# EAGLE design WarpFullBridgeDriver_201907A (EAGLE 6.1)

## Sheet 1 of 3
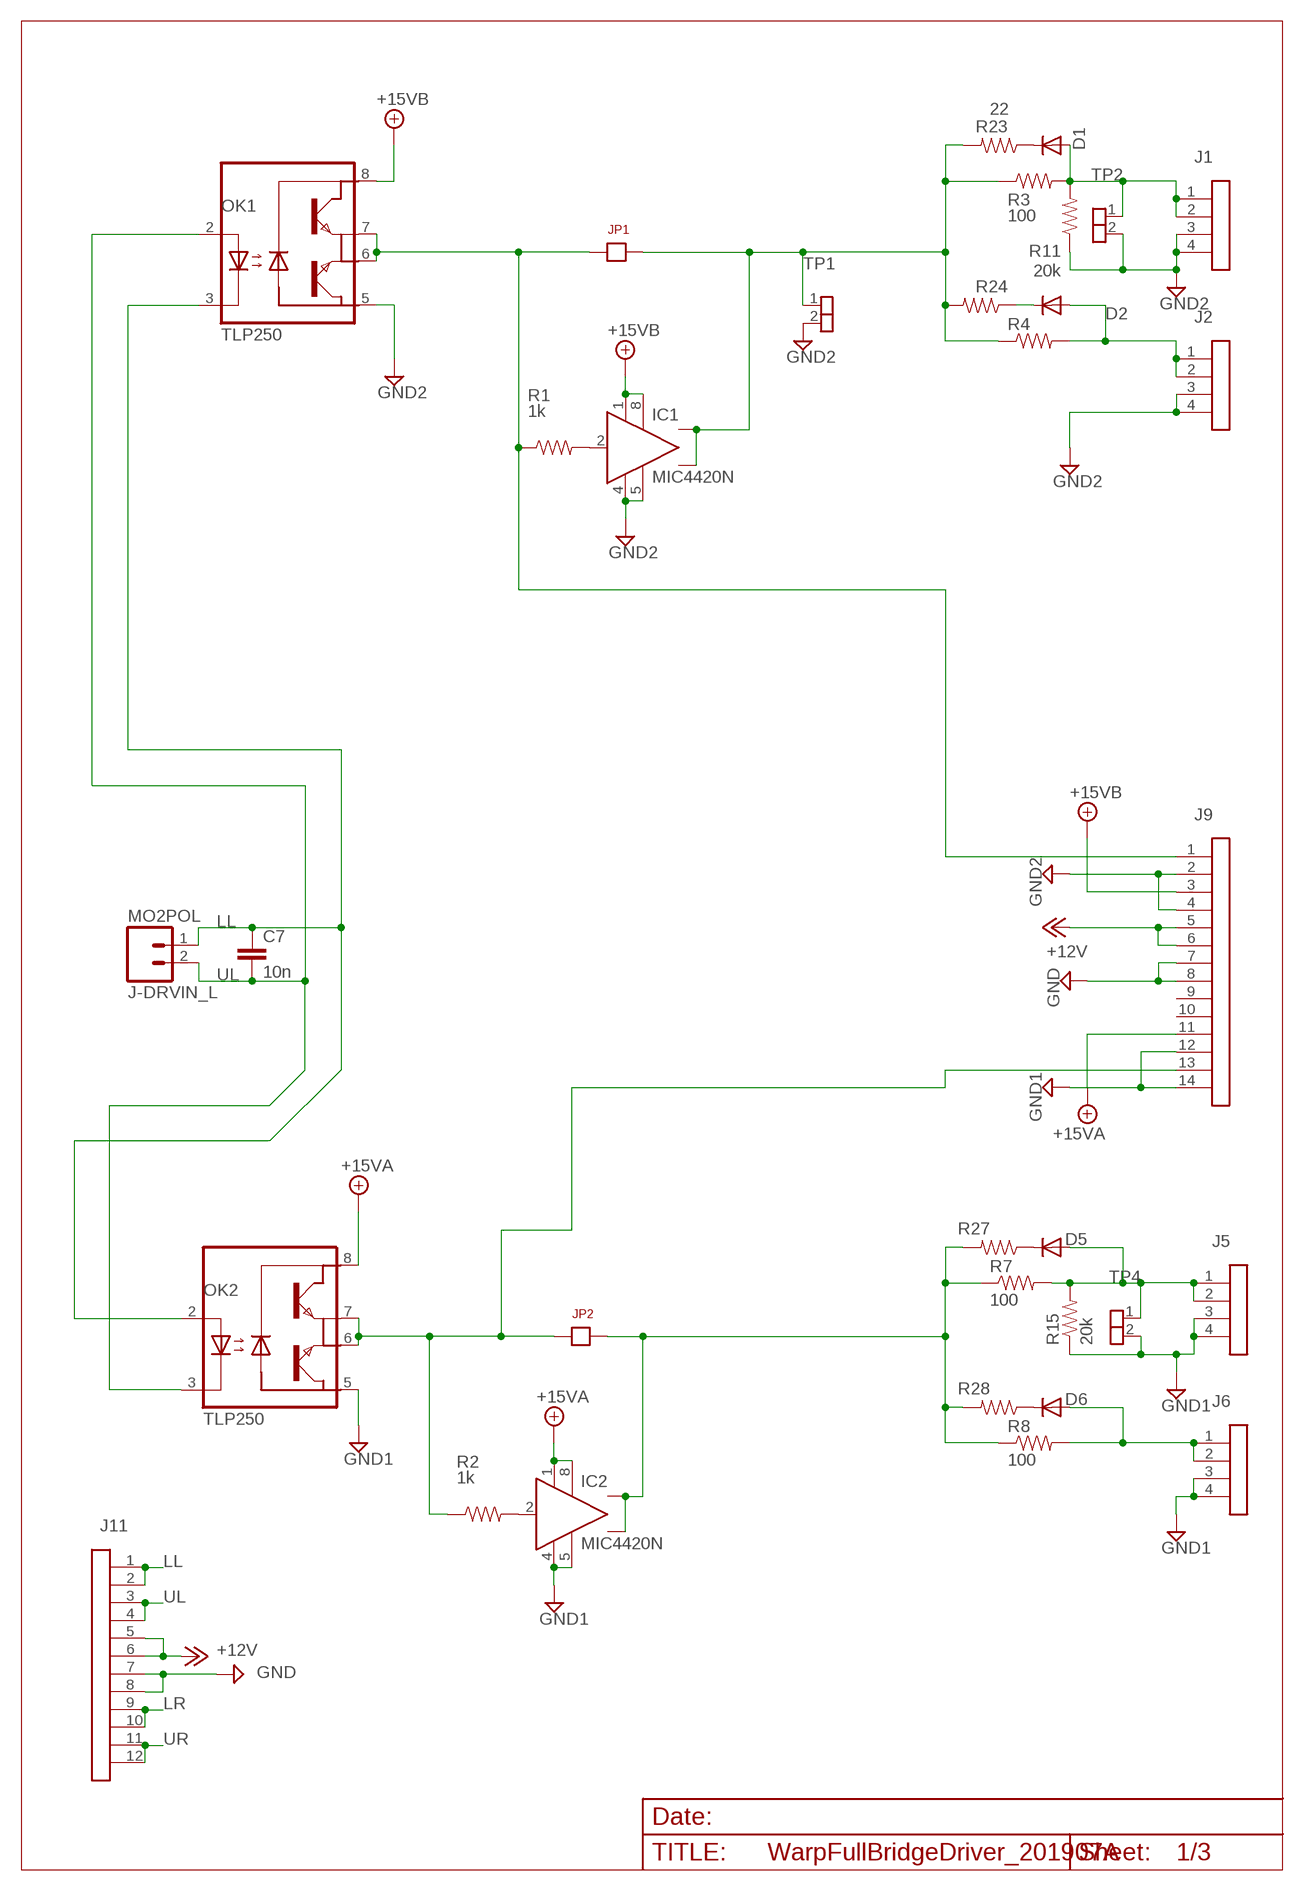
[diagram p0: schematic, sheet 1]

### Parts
C7  10n  BCAP  [BCAP]
D1  1N4148DO35-7  [D3]
D2  1N4148DO35-7  [D3]
D5  1N4148DO35-7  [D3]
D6  1N4148DO35-7  [D3]
IC1  MIC4420N  [DIL08]
IC2  MIC4420N  [DIL08]
J1  IDC04  [IDC04]
J2  IDC04  [IDC04]
J5  IDC04  [IDC04]
J6  IDC04  [IDC04]
J9  IDC14_LSPECIAL1  [IDC14-SPECIAL]
J11  IDC12  [IDC12]
J-DRVIN_L  MO2POL  [MOLEX-1X2]
JP1  JP1  [JP1]
JP2  JP1  [JP1]
OK1  TLP250  TLP250DIP8-L39  [DIL08-L39]
OK2  TLP250  TLP250DIP8-L39  [DIL08-L39]
R1  1k  RESISTORPTH-1/4W  [AXIAL-0.4]
R2  1k  RESISTORPTH-1/4W  [AXIAL-0.4]
R3  100  RESISTORPTH-1/4W  [AXIAL-0.4]
R4  100  RESISTORPTH-1/4W  [AXIAL-0.4]
R7  100  RESISTORPTH-1/4W  [AXIAL-0.4]
R8  100  RESISTORPTH-1/4W  [AXIAL-0.4]
R11  20k  R4  [AXIAL-0.4]
R15  20k  R4  [AXIAL-0.4]
R23  22  R4  [AXIAL-0.4]
R24  22  R4  [AXIAL-0.4]
R27  22  R4  [AXIAL-0.4]
R28  22  R4  [AXIAL-0.4]
TP1  SIL-2  [JP1]
TP2  SIL-2  [JP1]
TP4  SIL-2  [JP1]

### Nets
+12V: J9.5 J9.6 J11.5 J11.6 ; also sheet 2,3
+15VA: IC2.1(VS) IC2.8(VS1) J9.11 OK2.8(VCC) ; also sheet 3
+15VB: IC1.1(VS) IC1.8(VS1) J9.3 OK1.8(VCC) ; also sheet 3
GND: J9.7 J9.8 J11.7 J11.8 ; also sheet 2,3
GND1: IC2.4(GND) IC2.5(GND1) J5.3 J5.4 J6.3 J6.4 J9.12 J9.14 OK2.5(GND) R15.P$1 TP4.2 ; also sheet 3
GND2: IC1.4(GND) IC1.5(GND1) J1.3 J1.4 J2.3 J2.4 J9.2 J9.4 OK1.5(GND) R11.P$1 TP1.2 TP2.2 ; also sheet 3
LL: C7.1 J11.1 J11.2 J-DRVIN_L.1 OK1.3(C) OK2.2(A)
LR: J11.9 J11.10 ; also sheet 2
N$2: D2.A J2.1 J2.2 R4.P$2
N$3: D1.A J1.1 J1.2 R3.P$2 R11.P$2 TP2.1
N$4: D1.C R23.P$1
N$5: IC1.2(IN) R1.P$2
N$7: IC2.2(IN) R2.P$2
N$8: D6.A J6.1 J6.2 R8.P$2
N$12: D5.A J5.1 J5.2 R7.P$2 R15.P$2 TP4.1
N$17: IC1.6(OUT) IC1.7(OUT) JP1.2 R3.P$1 R4.P$1 R23.P$2 R24.P$2 TP1.1
N$18: J9.1 JP1.1 OK1.6(VO) OK1.7(VO2) R1.P$1
N$19: IC2.6(OUT) IC2.7(OUT) JP2.2 R7.P$1 R8.P$1 R27.P$2 R28.P$2
N$21: D2.C R24.P$1
N$22: J9.13 JP2.1 OK2.6(VO) OK2.7(VO2) R2.P$1
N$28: D5.C R27.P$1
N$31: D6.C R28.P$1
UL: C7.2 J11.3 J11.4 J-DRVIN_L.2 OK1.2(A) OK2.3(C)
UR: J11.11 J11.12 ; also sheet 2
Unconnected: J9.9 J9.10

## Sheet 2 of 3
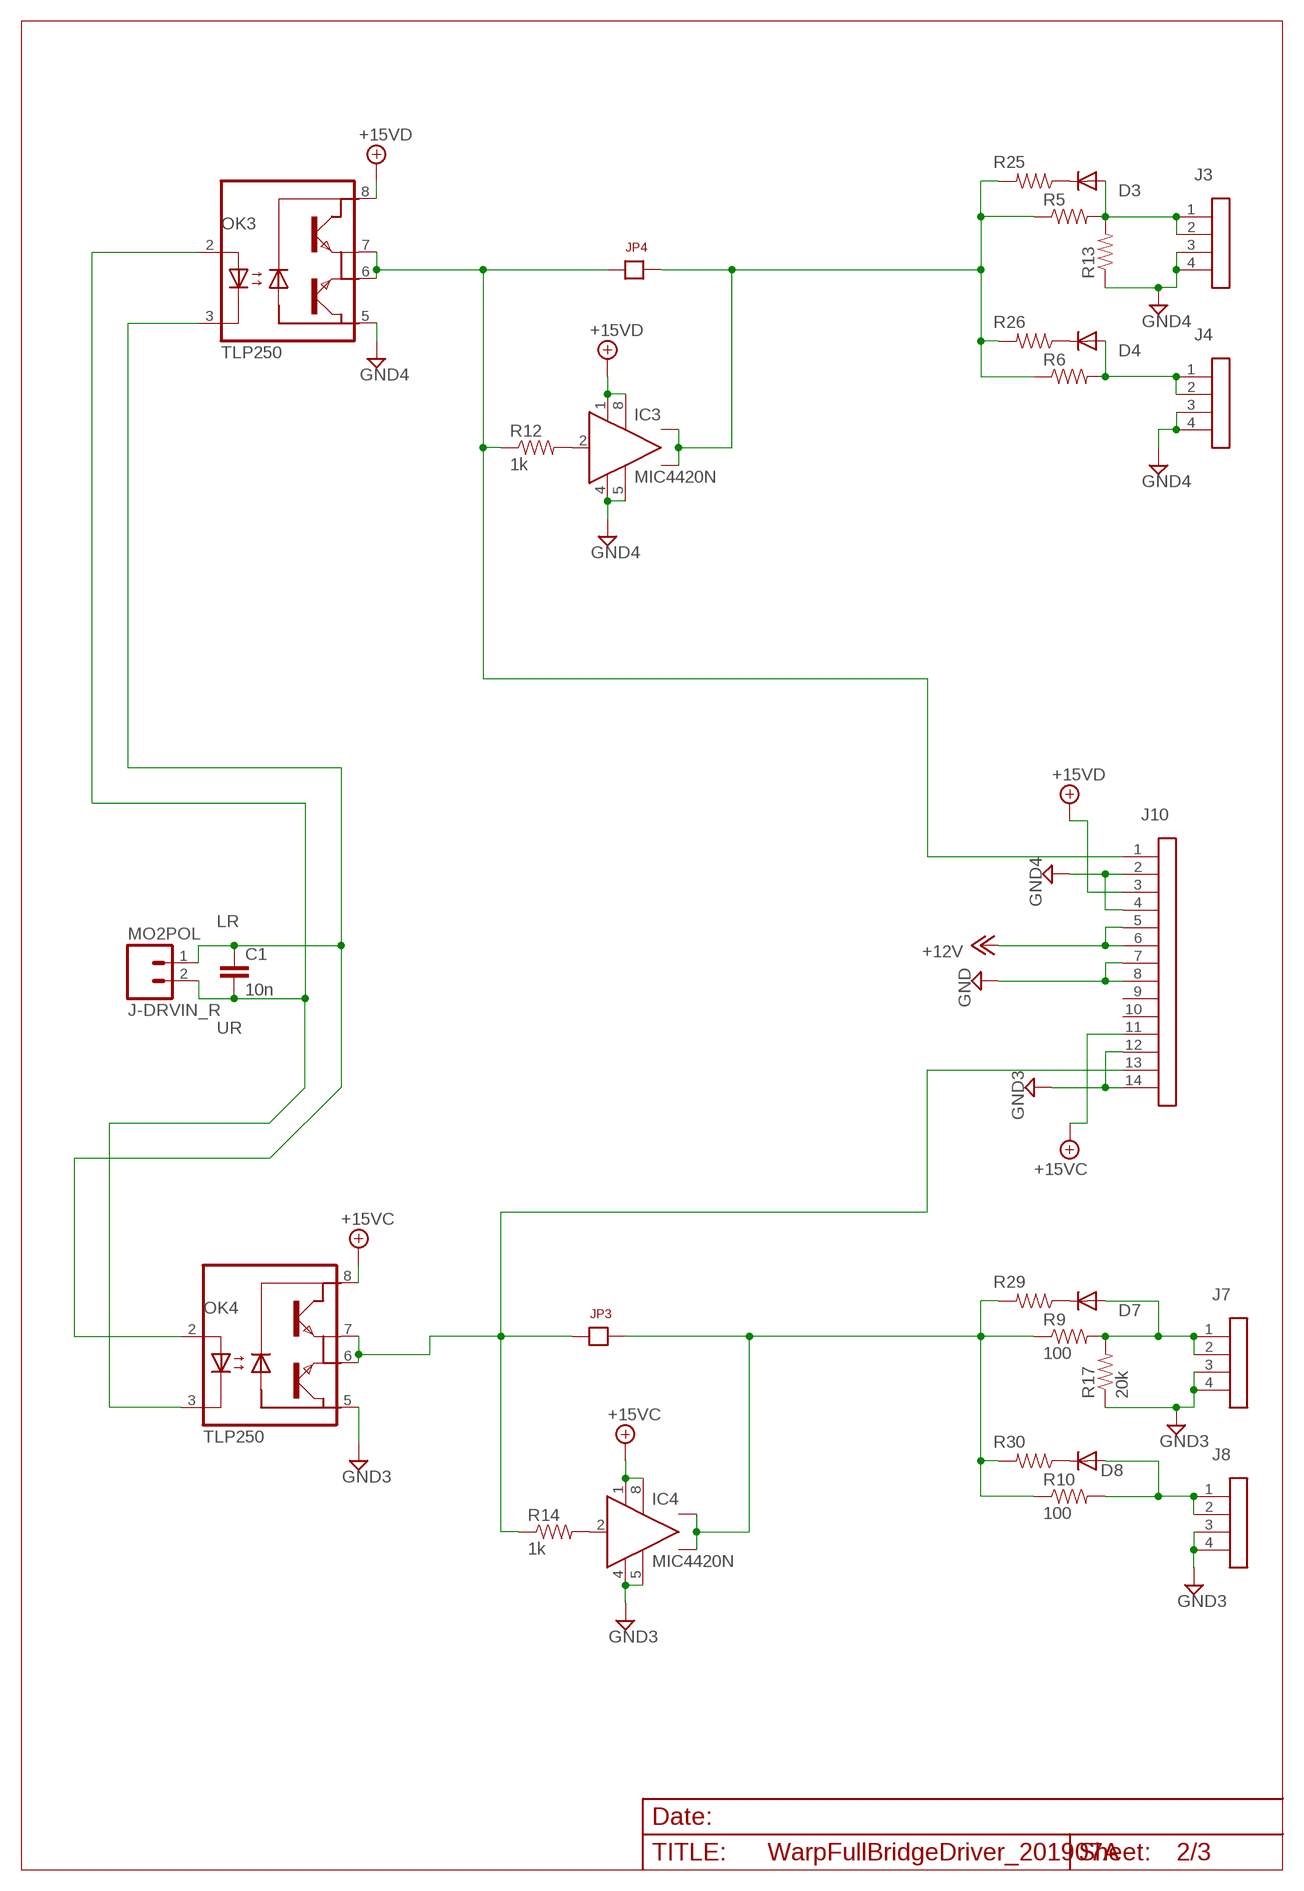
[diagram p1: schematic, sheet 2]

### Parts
C1  10n  BCAP  [BCAP]
D3  1N4148DO35-7  [D3]
D4  1N4148DO35-7  [D3]
D7  1N4148DO35-7  [D3]
D8  1N4148DO35-7  [D3]
IC3  MIC4420N  [DIL08]
IC4  MIC4420N  [DIL08]
J3  IDC04  [IDC04]
J4  IDC04  [IDC04]
J7  IDC04  [IDC04]
J8  IDC04  [IDC04]
J10  IDC14_LSPECIAL1  [IDC14-SPECIAL]
J-DRVIN_R  MO2POL  [MOLEX-1X2]
JP3  JP1  [JP1]
JP4  JP1  [JP1]
OK3  TLP250  TLP250DIP8-L39  [DIL08-L39]
OK4  TLP250  TLP250DIP8-L39  [DIL08-L39]
R5  100  RESISTORPTH-1/4W  [AXIAL-0.4]
R6  100  RESISTORPTH-1/4W  [AXIAL-0.4]
R9  100  RESISTORPTH-1/4W  [AXIAL-0.4]
R10  100  RESISTORPTH-1/4W  [AXIAL-0.4]
R12  1k  R4  [AXIAL-0.4]
R13  20k  R4  [AXIAL-0.4]
R14  1k  R4  [AXIAL-0.4]
R17  20k  R4  [AXIAL-0.4]
R25  22  R4  [AXIAL-0.4]
R26  22  R4  [AXIAL-0.4]
R29  22  R4  [AXIAL-0.4]
R30  22  R4  [AXIAL-0.4]

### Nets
+12V: J10.5 J10.6 ; also sheet 1,3
+15VC: IC4.1(VS) IC4.8(VS1) J10.11 OK4.8(VCC) ; also sheet 3
+15VD: IC3.1(VS) IC3.8(VS1) J10.3 OK3.8(VCC) ; also sheet 3
GND: J10.7 J10.8 ; also sheet 1,3
GND3: IC4.4(GND) IC4.5(GND1) J7.3 J7.4 J8.3 J8.4 J10.12 J10.14 OK4.5(GND) R17.P$1 ; also sheet 3
GND4: IC3.4(GND) IC3.5(GND1) J3.3 J3.4 J4.3 J4.4 J10.2 J10.4 OK3.5(GND) R13.P$1 ; also sheet 3
LR: C1.1 J-DRVIN_R.1 OK3.3(C) OK4.2(A) ; also sheet 1
N$1: IC3.6(OUT) IC3.7(OUT) JP4.2 R5.P$1 R6.P$1 R25.P$2 R26.P$2
N$6: IC4.6(OUT) IC4.7(OUT) JP3.2 R9.P$1 R10.P$1 R29.P$2 R30.P$2
N$9: D3.A J3.1 J3.2 R5.P$2 R13.P$2
N$10: D4.A J4.1 J4.2 R6.P$2
N$11: IC3.2(IN) R12.P$2
N$13: D7.A J7.1 J7.2 R9.P$2 R17.P$2
N$14: D8.A J8.1 J8.2 R10.P$2
N$15: J10.1 JP4.1 OK3.6(VO) OK3.7(VO2) R12.P$1
N$16: IC4.2(IN) R14.P$2
N$24: D3.C R25.P$1
N$25: D4.C R26.P$1
N$33: J10.13 JP3.1 OK4.6(VO) OK4.7(VO2) R14.P$1
N$34: D7.C R29.P$1
N$37: D8.C R30.P$1
UR: C1.2 J-DRVIN_R.2 OK3.2(A) OK4.3(C) ; also sheet 1
Unconnected: J10.9 J10.10

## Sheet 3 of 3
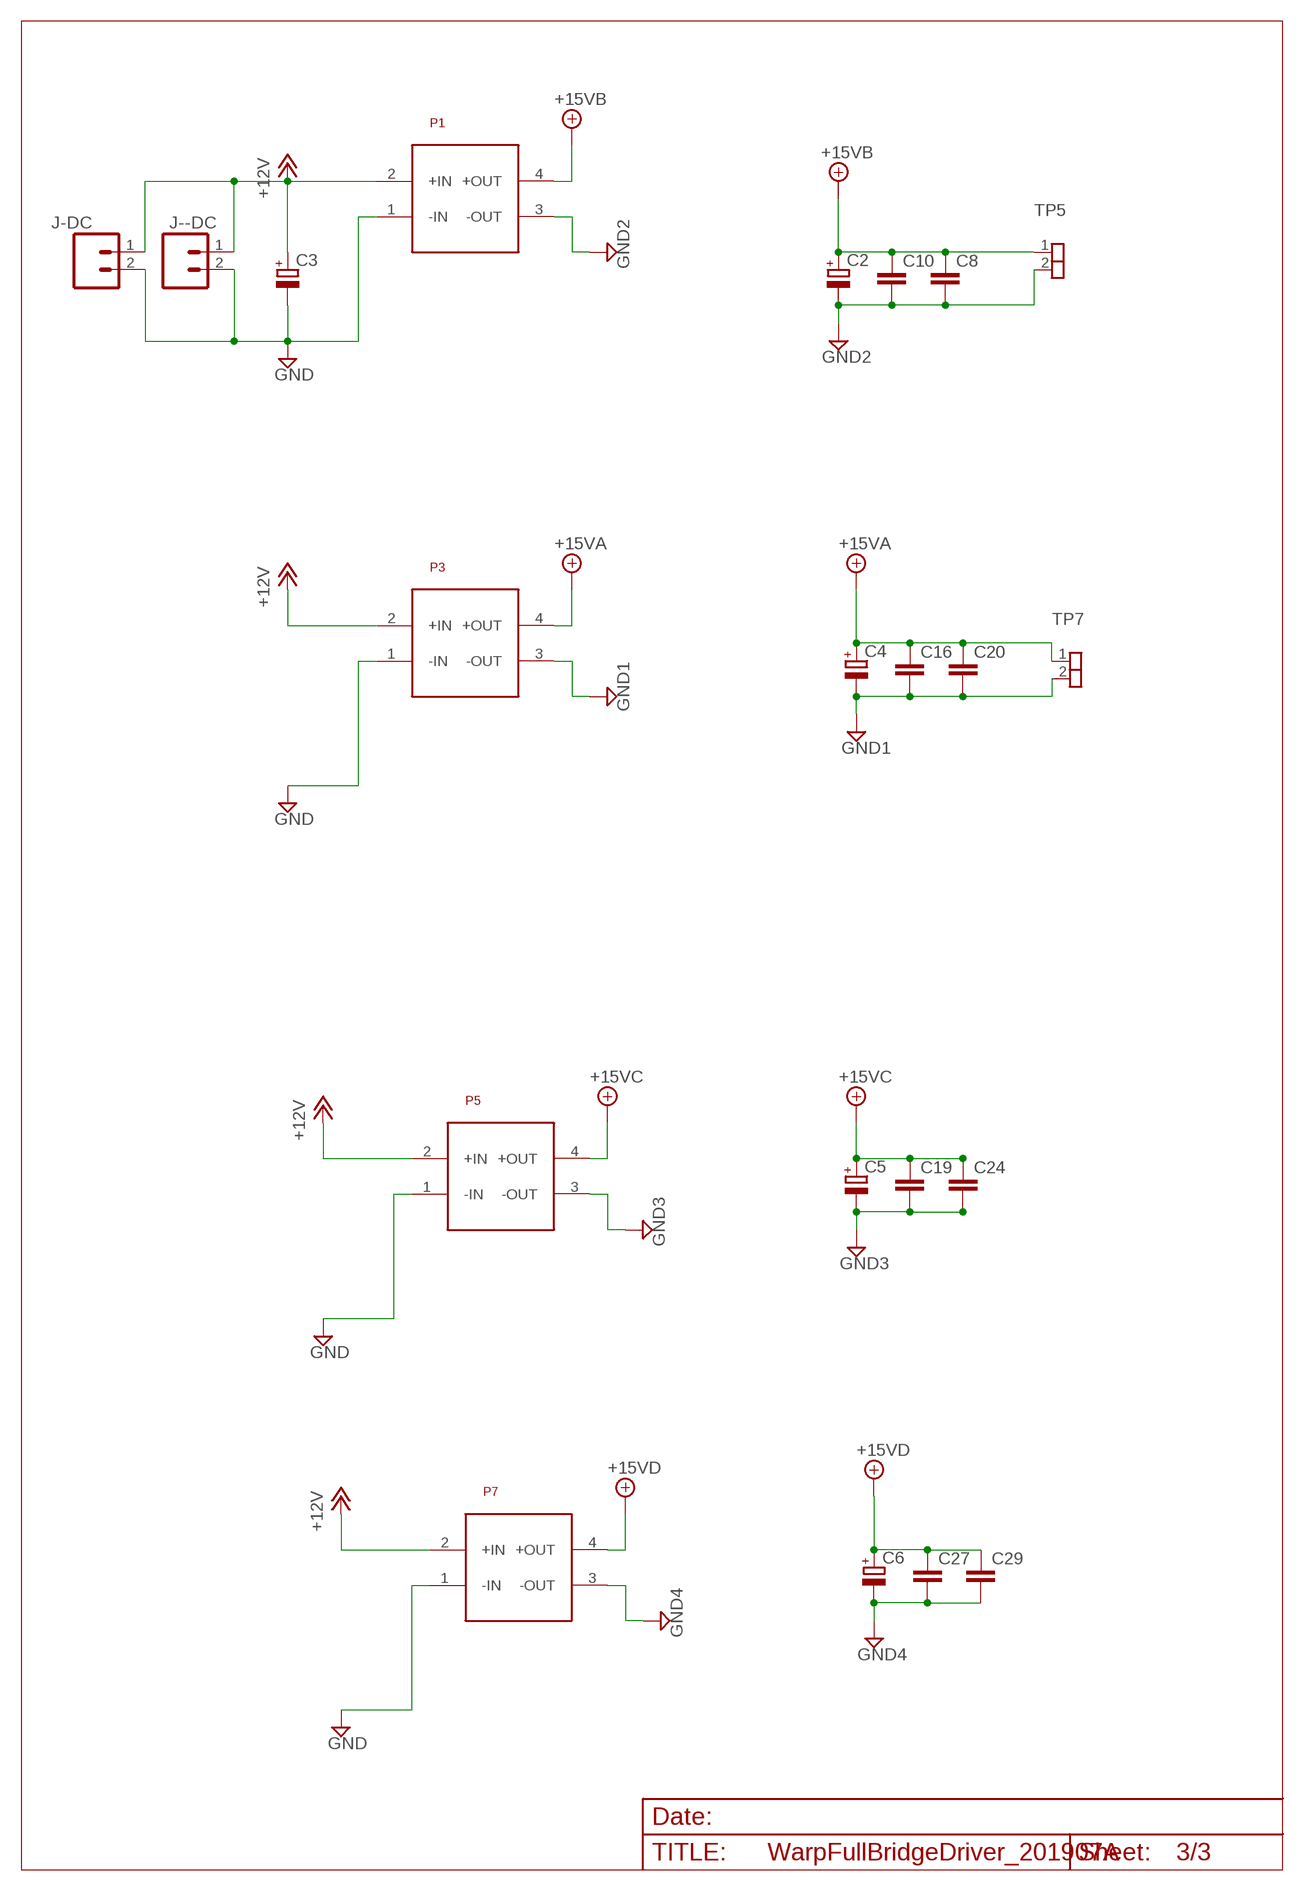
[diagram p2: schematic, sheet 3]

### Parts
C2  CPOL-EUE2.5-6  [E2,5-6]
C3  CPOL-EUE2.5-6  [E2,5-6]
C4  CPOL-EUE2.5-6  [E2,5-6]
C5  CPOL-EUE2.5-6  [E2,5-6]
C6  CPOL-EUE2.5-6  [E2,5-6]
C8  BCAP  [BCAP]
C10  BCAP  [BCAP]
C16  BCAP  [BCAP]
C19  BCAP  [BCAP]
C20  BCAP  [BCAP]
C24  BCAP  [BCAP]
C27  BCAP  [BCAP]
C29  BCAP  [BCAP]
J--DC  MO2POL  [MOLEX-1X2]
J-DC  MO2POL  [MOLEX-1X2]
P1  VBSD1-S12-S5  [VBSD1]
P3  VBSD1-S12-S5  [VBSD1]
P5  VBSD1-S12-S5  [VBSD1]
P7  VBSD1-S12-S5  [VBSD1]
TP5  SIL-2  [JP1]
TP7  SIL-2  [JP1]

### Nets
+12V: C3.+ J--DC.1 J-DC.1 P1.2(+IN) P3.2(+IN) P5.2(+IN) P7.2(+IN) ; also sheet 1,2
+15VA: C4.+ C16.1 C20.1 P3.4(+OUT) TP7.1 ; also sheet 1
+15VB: C2.+ C8.1 C10.1 P1.4(+OUT) TP5.1 ; also sheet 1
+15VC: C5.+ C19.1 C24.1 P5.4(+OUT) ; also sheet 2
+15VD: C6.+ C27.1 C29.1 P7.4(+OUT) ; also sheet 2
GND: C3.- J--DC.2 J-DC.2 P1.1(-IN) P3.1(-IN) P5.1(-IN) P7.1(-IN) ; also sheet 1,2
GND1: C4.- C16.2 C20.2 P3.3(-OUT) TP7.2 ; also sheet 1
GND2: C2.- C8.2 C10.2 P1.3(-OUT) TP5.2 ; also sheet 1
GND3: C5.- C19.2 C24.2 P5.3(-OUT) ; also sheet 2
GND4: C6.- C27.2 C29.2 P7.3(-OUT) ; also sheet 2

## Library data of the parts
C1 C7 C8 C10 C16 C19 C20 C24 C27 C29 = Andrew Misc:BCAP
C2-C6 = rcl:CPOL-EU: POLARIZED CAPACITOR, European symbol
D1-D8 = Andrew Misc:1N4148: DIODE
IC1-IC4 = Andrew IC:MIC4420: 6A-Peak Low-Side MOSFET Driver Bipolar/CMOS/DMOS Process http://www.micrel.com/_PDF/mic4420.pdf
J1-J8 = Andrew_Connectors:IDC04
J9 J10 = Andrew_Connectors:IDC14_L
J11 = Andrew_Connectors:IDC12
J--DC J-DC J-DRVIN_L J-DRVIN_R = Andrew_Connectors:MO2POL
JP1-JP4 = Andrew_Connectors:JP1
OK1-OK4 = Andrew IC:TLP250: HEWLETT PACKARD OPTO COUPLER
P1 P3 P5 P7 = Andrew ISOPWR:VBSD1-S12-S5
R1-R10 = SparkFun-Passives:RESISTOR: Resistor
R11-R15 R17 R23-R30 = Andrew Misc:R4
TP1 TP2 TP4 TP5 TP7 = Andrew_Connectors:SIL-2

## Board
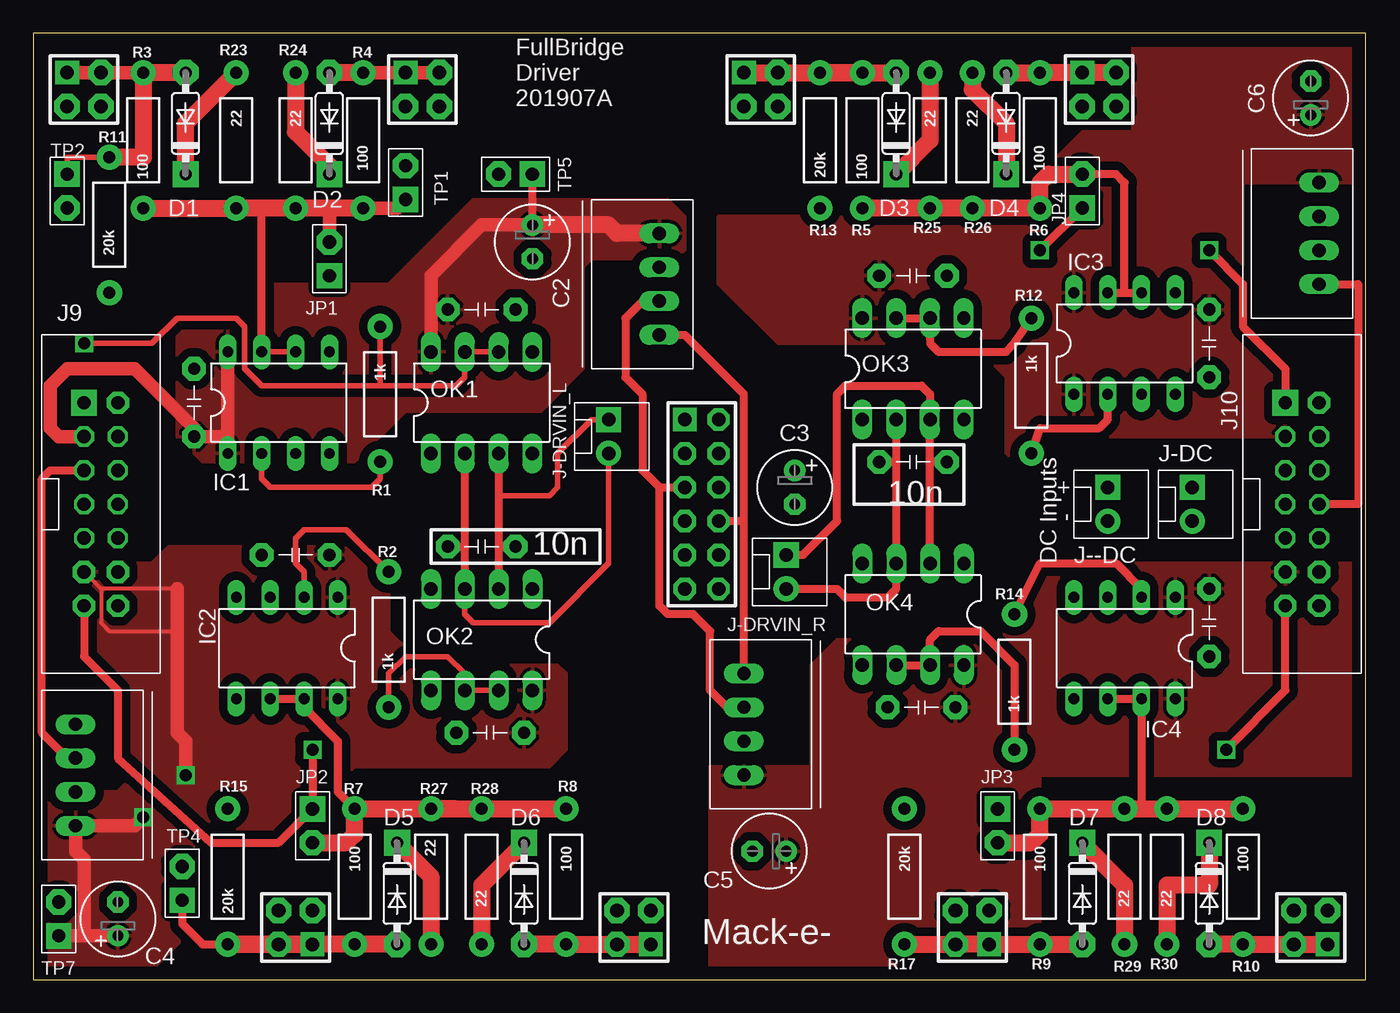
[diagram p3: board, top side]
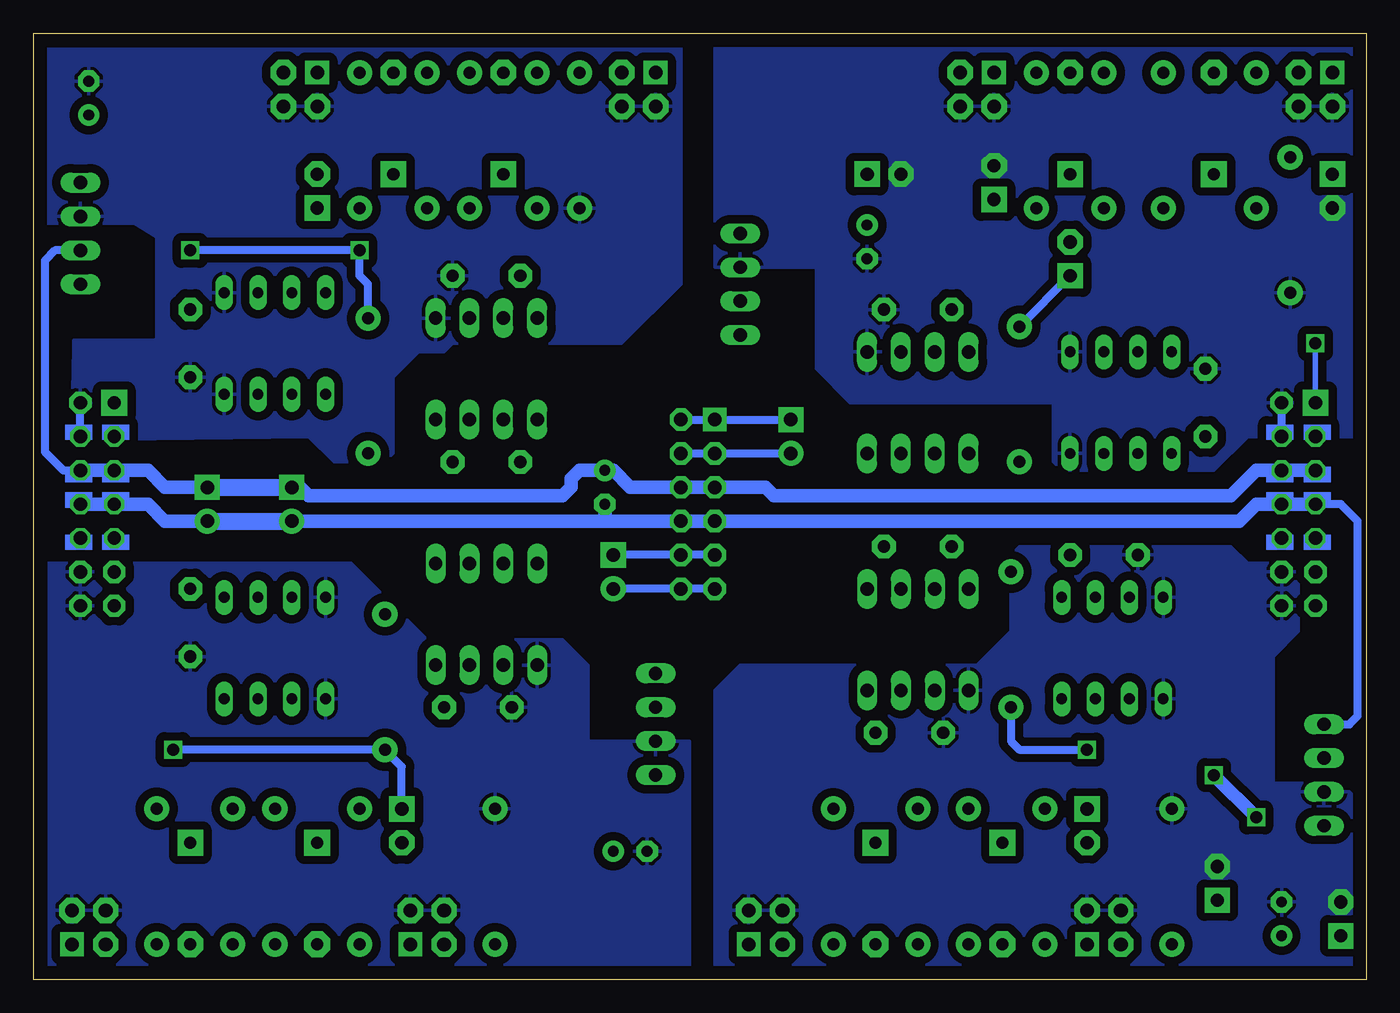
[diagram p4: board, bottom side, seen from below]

Size 100 x 71 mm. Coordinates in mm from the lower left corner, seen from the top.
Outline: 0,0 100,0 100,71 0,71 0,0
Copper layers (1*16): Top 0.035mm / dielectric 1.5mm / Bottom 0.035mm
Design rules: minimum track width 10mil, minimum drill 24mil, track to track 8mil, track to pad 8mil, pad to pad 8mil, via to via 8mil, smd to smd 8mil, copper to edge 40mil, drill to drill 8mil, minimum pad ring 10mil, minimum via ring 8mil, stop-mask expansion 4mil, vias tented up to drill 0mil, thermal gap 10mil

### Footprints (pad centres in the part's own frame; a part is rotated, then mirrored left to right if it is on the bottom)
BCAP = drill 0.914 pad 1.778 octagon: 1 -2.54,0; 2 2.54,0
E2,5-6 = drill 0.813 pad 1.6: + -1.27,0 | drill 0.813 pad 1.6 octagon: - 1.27,0
D3 = drill 0.914 pad 1.93 octagon: A 3.81,0 | drill 0.914 pad 1.93 square: C -3.81,0
DIL08 = drill 0.813 long: 1 -3.81,-3.81; 2 -1.27,-3.81; 3 1.27,-3.81; 4 3.81,-3.81; 5 3.81,3.81; 6 1.27,3.81; 7 -1.27,3.81; 8 -3.81,3.81
IDC04 = drill 1.016 pad 1.778 square: 1 -1.27,1.27 | drill 1.016 pad 1.905 octagon: 2 1.27,1.27; 3 -1.27,-1.27; 4 1.27,-1.27
IDC14-SPECIAL = drill 1 pad 1.93 square: 1 0,0 | drill 1 pad 1.676 octagon: 2 0,2.54; 11 12.7,0; 12 12.7,2.54; 13 15.24,0; 14 15.24,2.54 | drill 1 pad 1.143 octagon: 3 2.54,0; 4 2.54,2.54; 5 5.08,0; 6 5.08,2.54; 7 7.62,0; 8 7.62,2.54; 9 10.16,0; 10 10.16,2.54
IDC12 = drill 1.016 pad 1.778 square: 1 -1.27,6.35 | drill 1.016 pad 1.676 octagon: 2 1.27,6.35; 3 -1.27,3.81; 4 1.27,3.81; 5 -1.27,1.27; 6 1.27,1.27; 7 -1.27,-1.27; 8 1.27,-1.27; 9 -1.27,-3.81; 10 1.27,-3.81; 11 -1.27,-6.35; 12 1.27,-6.35
MOLEX-1X2 = drill 1.016 pad 1.88 square: 1 0,0 | drill 1.016 pad 1.88: 2 2.54,0
JP1 = drill 1 pad 1.905 square: 1 -1.27,0 | drill 1 pad 1.905 octagon: 2 1.27,0
DIL08-L39 = drill 1 long: 1 -3.81,-3.81; 2 -1.27,-3.81; 3 1.27,-3.81; 4 3.81,-3.81; 5 3.81,3.81; 6 1.27,3.81; 7 -1.27,3.81; 8 -3.81,3.81
VBSD1 = drill 1 long: 1 -3.81,0; 2 -1.27,0; 3 1.27,0; 4 3.81,0
AXIAL-0.4 = drill 0.9 pad 1.88: P$1 -5.08,0; P$2 5.08,0

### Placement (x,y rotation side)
C1  66.04,38.84 180 top
C2  37.47,55.35 270 top
C3  57.15,36.94 270 top
C4  6.35,4.55 90 top
C5  55.24,9.63 180 top
C6  95.89,66.14 90 top
C7  33.66,32.49 180 top
C8  12.06,43.28 90 top
C10  33.66,50.27 0 top
C16  34.29,18.52 180 top
C19  88.27,26.77 270 top
C20  19.68,31.85 180 top
C24  66.67,20.42 180 top
C27  88.27,47.73 270 top
C29  66.04,52.81 0 top
D1  11.43,64.24 90 top
D2  22.23,64.24 90 top
D3  64.77,64.24 90 top
D4  73.03,64.24 90 top
D5  27.3,6.45 270 top
D6  36.83,6.45 270 top
D7  78.74,6.45 270 top
D8  88.27,6.45 270 top
IC1  18.41,43.28 0 top
IC2  19.05,24.87 180 top
IC3  81.92,47.73 0 top
IC4  81.92,24.87 180 top
J1  3.81,66.78 0 top
J2  29.21,66.78 0 top
J3  54.61,66.78 0 top
J4  80.01,66.78 0 top
J5  19.68,3.91 180 top
J6  45.09,3.91 180 top
J7  70.48,3.91 180 top
J8  95.89,3.91 180 top
J9  3.81,43.28 270 top
J10  93.98,43.28 270 top
J11  50.16,35.66 0 top
J--DC  80.64,36.94 270 top
J-DC  87,36.94 270 top
J-DRVIN_L  43.18,42.02 270 top
J-DRVIN_R  56.52,31.85 270 top
JP1  22.23,54.08 90 top
JP2  20.95,11.54 270 top
JP3  72.39,11.54 270 top
JP4  78.74,59.16 90 top
OK1  33.66,43.28 0 top
OK2  33.66,25.51 180 top
OK3  66.04,45.83 0 top
OK4  66.04,27.41 180 top
P1  46.99,52.17 90 top
P3  3.17,15.34 270 top
P5  53.34,19.16 270 top
P7  96.52,55.98 90 top
R1  26.04,43.92 270 top
R2  26.67,25.51 90 top
R3  8.26,62.97 90 top
R4  24.77,62.97 90 top
R5  62.23,62.97 90 top
R6  75.56,62.97 90 top
R7  24.13,7.73 270 top
R8  40.01,7.73 270 top
R9  75.56,7.73 270 top
R10  90.81,7.73 270 top
R11  5.71,56.62 90 top
R12  74.93,44.55 270 top
R13  59.05,62.97 90 top
R14  73.66,22.33 90 top
R15  14.61,7.73 270 top
R17  65.41,7.73 270 top
R23  15.24,62.97 270 top
R24  19.68,62.97 270 top
R25  67.31,62.97 270 top
R26  70.48,62.97 270 top
R27  29.84,7.73 90 top
R28  33.66,7.73 90 top
R29  81.92,7.73 90 top
R30  85.09,7.73 90 top
TP1  27.94,59.8 90 top
TP2  2.54,59.16 270 top
TP4  11.18,7.22 90 top
TP5  36.2,60.43 180 top
TP7  1.91,4.55 90 top

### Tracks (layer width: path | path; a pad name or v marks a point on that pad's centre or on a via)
+12V
  Top 0.61: P1.2 45.72,50.91 44.45,49.64 44.45,45.19 45.72,43.92 45.72,38.2 46.99,36.94 | 46.99,36.94 J11.5 | P3.2 2.54,16.61 0.64,18.52 0.64,37.57 1.27,38.2 J9.5 | P5.2 52.07,20.42 50.8,21.7 50.8,26.14 49.53,27.41 47.62,27.41 46.99,28.05 46.99,36.94
  Bottom 0.61: P7.2 98.42,54.72 99.19,53.95 99.19,39.6 97.79,38.2 J10.6
  Bottom 1.016: J10.6 J10.5 91.44,38.2 90.17,36.94 J-DC.1 | J9.5 J9.6 8.26,38.2 10.16,36.3 44.45,36.3 45.09,36.94 J11.5 J11.6 55.24,36.94 56.52,38.2 C3.+ 59.05,38.2 59.69,37.57 59.69,36.94 60.33,36.3 79.38,36.3 80.01,36.94 J--DC.1
  Bottom 1.27: J-DC.1 J--DC.1
+15VA  (via drill 0.9)
  Top 0.305: 10.79,29.31 5.08,29.31 | J9.11 5.08,29.31 | 5.08,29.31 5.08,26.77 5.71,26.14 10.79,26.14
  Top 1.016: C4.+ 3.81,3.28 | TP7.1 3.81,3.28 | 3.81,3.28 3.81,9 3.17,9.63 P3.4 7.62,11.54 v8.26,12.17 | v11.43,15.34 11.43,17.88 10.79,18.52 10.79,26.14 10.79,29.31
  Bottom 1.016: v8.26,12.17 v11.43,15.34
  pour Top (isolate 0.635): 0.64,12.8 0.64,13.44 1.27,14.07 6.35,14.07 6.99,14.71 6.99,22.33 4.45,24.87 4.45,30.59 5.08,31.22 8.89,31.22 10.16,32.49 26.04,32.49 26.67,31.85 26.67,26.14 29.21,23.6 39.37,23.6 40.01,22.97 40.01,17.25 38.73,15.98 24.13,15.98 8.89,0.74 0.64,0.74
+15VB
  Top 0.61: C2.+ TP5.1
  Top 1.016: C2.+ 33.66,56.62 29.84,52.81 OK1.8 | IC1.8 14.61,40.74 | 14.61,40.74 IC1.1 | 14.61,40.74 C8.1 12.06,41.38 7.62,45.83 2.54,45.83 1.27,44.55 1.27,41.38 1.91,40.74 J9.3
  Top 1.27: P1.4 43.81,55.98 43.18,56.62 C2.+
  pour Top (isolate 0.635): 24.13,38.84 12.7,38.84 10.79,40.74 10.79,50.91 12.06,52.17 26.67,52.17 33.02,58.53 47.62,58.53 48.9,57.25 48.9,54.72 48.26,54.08 41.91,54.08 41.27,53.44 41.27,45.83 38.1,42.65 27.94,42.65
+15VC
  pour Top (isolate 0.635): 50.8,15.98 50.8,0.74 75.56,0.74 75.56,15.34 99.06,15.34 99.06,31.22 76.2,31.22 70.48,25.51 60.33,25.51 58.42,23.6 58.42,15.98
+15VD
  pour Top (isolate 0.635): 99.69,59.8 99.69,69.95 82.55,69.95 82.55,63.61 78.74,63.61 72.39,57.25 51.44,57.25 51.44,52.17 55.88,47.73 70.48,47.73 73.03,45.19 73.03,39.48 73.66,38.84 78.11,38.84 80.01,40.74 94.61,40.74 94.61,47.73 91.44,47.73 90.81,48.37 90.81,59.8
GND
  Top 0.61: P1.1 48.9,48.37 53.34,43.92 53.34,34.4 | 53.34,34.4 J11.8 | P5.1 53.34,34.4 | P7.1 99.44,52.17 99.44,35.66 J10.8
  Bottom 0.61: P3.1 1.27,19.16 0.64,19.79 0.64,34.4 1.91,35.66 J9.7
  Bottom 1.016: J9.7 J9.8 8.26,35.66 9.53,34.4 J11.7 J11.8 57.15,34.4 | J-DC.2 90.17,34.4 91.44,35.66 J10.7 J10.8 | J--DC.2 57.15,34.4 | C3.- 57.15,34.4
  Bottom 1.27: J-DC.2 J--DC.2
GND1
  pour Bottom (isolate 0.61): 0.64,0.74 48.9,0.74 48.9,21.7 46.99,23.6 29.21,23.6 26.67,26.14 26.67,31.85 26.04,32.49 10.16,32.49 8.89,31.22 5.08,31.22 5.08,26.14 6.99,24.23 6.99,14.71 1.91,14.71 0.64,13.44
GND2
  Bottom 0.61: J9.4 J9.2
  pour Bottom (isolate 0.635): 0.64,40.74 0.64,70.59 48.9,70.59 48.9,53.44 41.27,53.44 41.27,45.83 38.73,43.28 23.5,43.28 23.5,38.84 22.86,38.2 11.43,38.2 8.89,40.74
GND3
  pour Bottom (isolate 0.635): 50.8,17.88 50.8,0.74 99.06,0.74 99.06,31.22 76.2,31.22 70.48,25.51 60.33,25.51 58.42,23.6 58.42,17.88
GND4
  Bottom 0.61: J10.4 J10.2
  pour Bottom (isolate 0.635): 96.52,40.49 96.9,40.49 97.16,41 97.03,47.35 97.03,47.98 90.93,47.98 90.81,48.11 90.81,55.73 92.46,56.75 99.69,56.75 99.69,69.95 51.44,69.95 51.44,52.17 55.88,47.73 68.58,47.73 69.22,47.09 71.12,47.09 73.03,45.19 73.03,39.48 73.66,38.84 77.47,38.84 79.38,40.74
LL
  Top 0.406: 34.92,36.3 38.73,36.3 39.37,36.94 39.37,39.48 41.91,42.02 J-DRVIN_L.1
  Top 0.61: OK1.3 34.92,36.3 34.92,32.49 | 34.92,32.49 OK2.2 | C7.1 34.92,32.49
  Bottom 0.61: J11.2 J11.1 J-DRVIN_L.1
LR
  Top 0.61: OK4.2 67.31,38.84 | 67.31,38.84 OK3.3 67.31,43.92 66.67,44.55 60.96,44.55 60.33,43.92 60.33,34.4 57.78,31.85 J-DRVIN_R.1 | C1.1 67.31,38.84
  Bottom 0.61: J11.9 J11.10 J-DRVIN_R.1
N$1
  Top 0.61: 81.92,51.54 IC3.6 | IC3.7 81.92,51.54 | 81.92,51.54 81.92,59.8 81.28,60.43 JP4.2
  Top 1.27: R5.P$1 R25.P$2 R26.P$2 R6.P$1 75.56,59.8 76.2,60.43 JP4.2
N$2
  Top 1.016: R4.P$2 J2.1 J2.2
  Top 1.27: R4.P$2 D2.A
N$3
  Top 0.406: TP2.1 2.54,61.7 R11.P$2
  Top 1.016: R3.P$2 J1.2 J1.1
  Top 1.27: D1.A R3.P$2 8.26,61.7 R11.P$2
N$4
  Top 1.27: D1.C 11.43,64.24 R23.P$1
N$5
  Top 0.406: R1.P$2 26.04,37.57 25.4,36.94 17.78,36.94 17.14,37.57 IC1.2
N$6
  Top 0.61: IC4.6 IC4.7 83.19,12.8
  Top 1.27: R10.P$1 R30.P$2 83.19,12.8 R29.P$2 R9.P$1 75.56,10.9 74.93,10.27 JP3.2
N$7
  Top 0.406: R2.P$2 23.5,33.76 20.32,33.76 19.68,33.12 19.68,31.22 20.32,30.59 IC2.2
N$8
  Top 1.27: D6.A R8.P$2 J6.2 J6.1
N$9
  Top 1.27: J3.1 J3.2 R5.P$2 R13.P$2 D3.A
N$10
  Top 1.27: D4.A R6.P$2 J4.1 J4.2
N$11
  Top 0.61: R12.P$2 75.56,41.38 80.01,41.38 80.64,42.02 IC3.2
N$12
  Top 0.61: TP4.1 11.18,4.17 12.7,2.64 R15.P$2
  Top 1.27: D5.A R7.P$2 R15.P$2 J5.1 J5.2
N$13
  Top 1.27: D7.A R9.P$2 J7.1 J7.2 R17.P$2
N$14
  Top 1.27: D8.A R10.P$2 J8.2 J8.1
N$15  (via drill 0.9)
  Top 0.61: OK3.7 OK3.6 67.31,47.73 67.94,47.09 73.03,47.09 73.66,47.73 R12.P$1 | v88.27,54.72 90.81,52.17 90.81,49 93.98,45.83 J10.1 | v75.56,54.72 JP4.1
  Bottom 0.61: v88.27,54.72 v75.56,54.72 75.56,52.81 74.93,52.17 R12.P$1
N$16
  Top 0.61: R14.P$2 75.56,31.22 81.28,31.22 83.19,29.31 IC4.2
N$17
  Top 0.406: IC1.7 IC1.6
  Top 0.61: IC1.7 17.14,57.89
  Top 1.016: JP1.2 22.23,57.89 | TP1.1 27.3,57.89 R4.P$1
  Top 1.27: R4.P$1 22.23,57.89 R24.P$2 17.14,57.89 R23.P$2 R3.P$1
N$18  (via drill 0.9)
  Top 0.406: R1.P$1 26.04,44.55 | 26.04,44.55 31.75,44.55 32.38,45.19 OK1.7 OK1.6 | 26.04,44.55 17.14,44.55 15.88,45.83 15.88,49 15.24,49.64 10.79,49.64 8.89,47.73 v3.81,47.73
  Bottom 0.406: J9.1 v3.81,47.73
  Bottom 0.61: JP1.1 R1.P$1
N$19
  Top 0.61: IC2.6 IC2.7 20.32,20.42 22.86,17.88 22.86,14.07 R7.P$1
  Top 1.27: 31.75,12.8 R27.P$2 | R27.P$2 R28.P$2 R8.P$1 | R27.P$2 R7.P$1 24.13,10.9 23.5,10.27 JP2.2
N$21
  Top 1.27: R24.P$1 19.68,63.61 22.23,61.06 D2.C
N$22  (via drill 0.9)
  Top 0.406: OK2.7 OK2.6 32.38,22.97 31.11,24.23 27.94,24.23 26.67,22.97 R2.P$1
  Top 0.61: v20.95,17.25 JP2.1 18.41,10.27 13.34,10.27 6.35,16.61 6.35,21.7 3.81,24.23 J9.13
  Bottom 0.61: R2.P$1 26.67,17.88 26.04,17.25 v20.95,17.25
N$24
  Top 1.27: R25.P$1 67.31,62.97 D3.C
N$25
  Top 1.27: R26.P$1 70.48,66.78 73.03,64.24 D4.C
N$28
  Top 1.27: D5.C 29.84,7.73 R27.P$1
N$31
  Top 1.27: D6.C 33.66,7.09 R28.P$1
N$33  (via drill 0.9)
  Top 0.61: OK4.6 OK4.7 67.31,25.51 67.94,26.14 71.12,26.14 73.66,23.6 R14.P$1 | v89.53,17.25 93.98,21.7 J10.13
  Bottom 0.61: JP3.1 72.39,15.98 R14.P$1 v89.53,17.25
N$34
  Top 1.27: D7.C 81.92,7.09 R29.P$1
N$37
  Top 1.27: D8.C 88.27,7.09 85.09,7.09 R30.P$1
UL
  Top 0.406: J-DRVIN_L.2 43.18,31.22 38.73,26.77 33.02,26.77 32.38,27.41 OK2.3
  Top 0.61: OK1.2 32.38,32.49 | 32.38,32.49 OK2.3 | C7.2 32.38,32.49
  Bottom 0.61: J11.4 J11.3 J-DRVIN_L.2
UR
  Top 0.61: 64.77,38.84 OK4.3 64.77,29.31 64.14,28.68 60.96,28.68 60.33,29.31 J-DRVIN_R.2 | 64.77,38.84 OK3.2 | C1.2 64.77,38.84
  Bottom 0.61: J11.11 J11.12 J-DRVIN_R.2

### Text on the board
tPlace: FullBridge | Driver | 201907A | + | 10n | - | 10n | DC Inputs | Mack-e-

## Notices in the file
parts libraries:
SparkFun-Passives: Licensing: CC v3.0 Share-Alike You are welcome to use this library for commercial purposes.
